(* Logix 5000 AddOnInstructionDefinition export Banner_B25_B55_PD_v4; software revision 33.00 *)

TYPE Banner_B25_B55_PDI_v4 :   // Process Data for a B25 or B55. This will include event information.
STRUCT
   Output_State : SINT;   // 0 = Inactive, 1 = Active
   Alarm_State : SINT;   // 0 = Inactive, 1 = Active
   Signal_Level : SINT;   // Signal Mode - Signal places 100% at taught condition and 0% at no signal. Switchpoint Centric paces 100% at taught conditition and 50% at switchpoint.
END_STRUCT
END_TYPE

ADD_ON_INSTRUCTION Banner_B25_B55_PD_v4   (* revision 4.0, vendor Banner Engineering *)
// Take raw process data and convert it to usable values.
VAR_INPUT
   SINT0 : SINT; {required}
   SINT1 : SINT; {required}
END_VAR
VAR_IN_OUT
   PD : Banner_B25_B55_PDI_v4; {required}
END_VAR

ROUTINE Logic   (* ladder *)
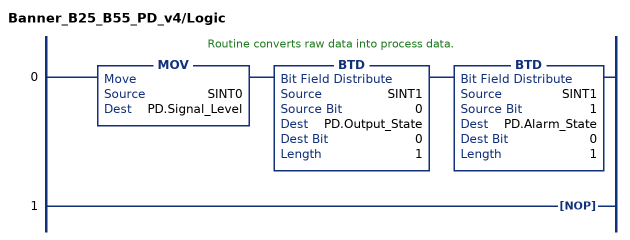
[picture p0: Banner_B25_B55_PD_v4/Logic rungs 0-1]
   // Routine converts raw data into process data.
   0: MOV(SINT0,PD.Signal_Level)BTD(SINT1,0,PD.Output_State,0,1)BTD(SINT1,1,PD.Alarm_State,0,1);
   1: NOP();
END_ROUTINE
END_ADD_ON_INSTRUCTION
